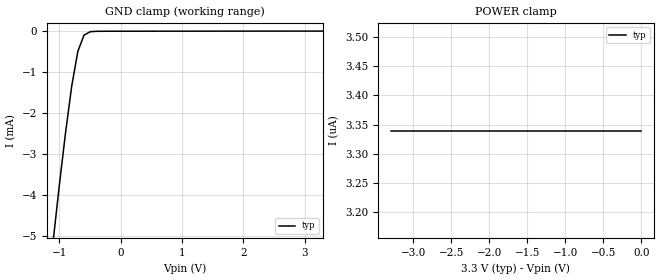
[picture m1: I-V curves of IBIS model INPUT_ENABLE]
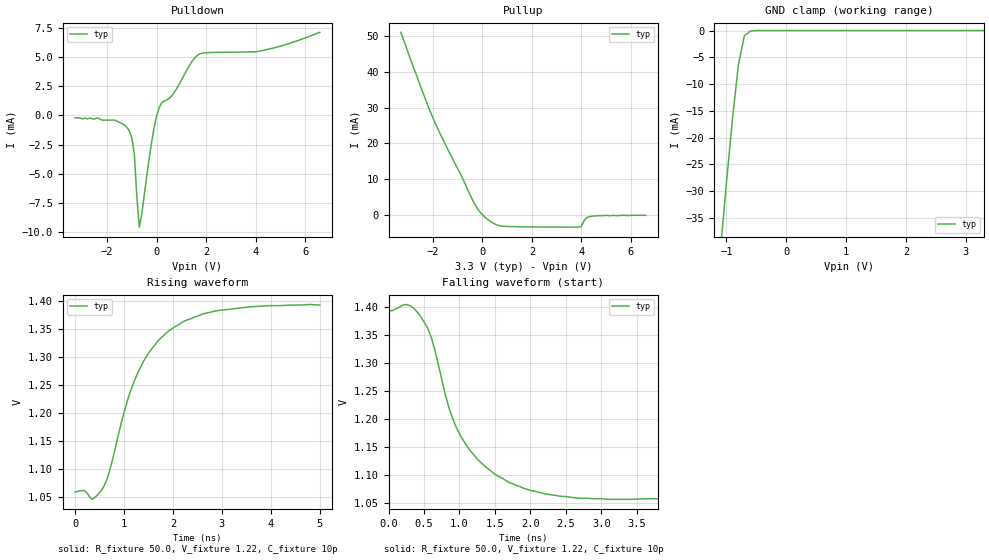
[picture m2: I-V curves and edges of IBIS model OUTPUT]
|   Texas Instruments Incorporated
|   Data Transmissions Products
|   IBIS Model for SN65LVDS389
|   38DBT TSSOP Package
[IBIS Ver]   2.1
[Comment char]   |_char
[File name]   lvds389.ibs
[File Rev]   1.0
[Date]   12Jan00
[Source]   File originated at Texas Instruments Incorporated.
   Data Transmission Products Group.
[Notes]   Model revved in Nov02 to fix common-mode bug  -TMF-
[Disclaimer]
(C) Copyright Texas Instruments Incorporated 2000
   All rights reserved
  Texas Instruments Incorporated hereby grants the user of this IBIS
model a non-exclusive, nontransferable license to use this IBIS model
under the following terms.  Before using this IBIS model, the user
should read this license.  If the user does not accept these terms,
the IBIS model should be returned to Texas Instruments within 30 days.
  The user is granted this license only to use the IBIS model and
is not granted rights to sell, load, rent, lease or license the IBIS
model in whole or in part, or in modified form to anyone other than
user.  User may modify the IBIS model to suit its specific applications
but rights to derivative works and such modifications shall belong to
Texas Instruments.
  This IBIS model is provided on an "AS IS" basis and Texas Instruments
makes absolutely no warranty with respect to the information contained
herein.  TEXAS INSTRUMENTS DISCLAIMS AND CUSTOMER WAIVES ALL WARRANTIES,
EXPRESS OR IMPLIED, INCLUDING WARRANTIES OF MERCHANTABILITY OR FITNESS
FOR A PARTICULAR PURPOSE. The entire risk as to quality and performance
is with the Customer. ACCORDINGLY, IN NO EVENT SHALL THE COMPANY BE LIABLE
FOR ANY DAMAGES, WHETHER IN CONTRACT OR TORT,INCLUDING ANY LOST PROFITS
OR OTHER INCIDENTAL, CONSEQUENTIAL, EXEMPLARY, OR PUNITIVE DAMAGES ARISING
OUT OF THE USE OR APPLICATION OF THE IBIS model provided in this package.
Further, Texas Instruments reserves the right to discontinue or make changes
without notice to any product herein to improve reliability, function, or
design. Texas Instruments does not convey any license under patent rights
or any other intellectual property rights, including those of third parties.
Contact Texas Instruments at ATTN:DATA TRANSMISSIONS
Thomas Fisher 12500 TI Boulevard, M/S 8710  Dallas, Texas 75243
[Copyright]   Copyright 2000, Texas Instruments, All Rights Reserved
[Component]   LVDS389DGG
[Manufacturer]  Texas Instruments Incorporated
[Package]
|   typ   min   max
R_pkg   0.040   0.035   0.047
L_pkg   2.433nH   1.956nH   3.508nH
C_pkg   0.451pF   0.362pF   0.635pF
[Pin]   signal_name   model_name   R_pin   L_pin   C_pin
1   GND   GND   0.047   3.508n   0.598p
2   VCC   POWER   0.047   3.231n   0.634p
3   GND   GND   0.046   2.932n   0.570p
4   ENA   INPUT_ENABLE   0.043   2.459n   0.459p
5   A1A   INPUT_ENABLE   0.035   2.103n   0.387p
6   A2A   INPUT_ENABLE   0.036   2.005n   0.369p
7   A3A   INPUT_ENABLE   0.035   1.956n   0.365p
8   A4A   INPUT_ENABLE   0.036   1.965n   0.364p
9   GND   GND   0.036   1.965n   0.363p
10   VCC   POWER   0.036   1.974n   0.362p
11   GND   GND   0.036   1.965n   0.362p
12   B1A   INPUT_ENABLE   0.036   1.965n   0.364p
13   B2A   INPUT_ENABLE   0.036   1.956n   0.365p
14   B3A   INPUT_ENABLE   0.036   2.005n   0.369p
15   B4A   INPUT_ENABLE   0.035   2.102n   0.387p
16   ENB   INPUT_ENABLE   0.043   2.459n   0.459p
17   GND   GND   0.046   2.932n   0.570p
18   VCC   POWER   0.047   3.231n   0.634p
19   GND   GND   0.047   3.508n   0.598p
20   B4Z   OUTPUT   0.047   3.508n   0.598p
21   B4Y   OUTPUT   0.047   3.231n   0.634p
22   B3Z   OUTPUT   0.046   2.932n   0.570p
23   B3Y   OUTPUT   0.043   2.459n   0.458p
24   B2Z   OUTPUT   0.035   2.103n   0.387p
25   B2Y   OUTPUT   0.036   2.005n   0.369p
26   B1Z   OUTPUT   0.035   1.956n   0.365p
27   B1Y   OUTPUT   0.036   1.965n   0.364p
28   NC   NC
29   NC   NC
30   NC   NC
31   A4Z   OUTPUT   0.036   1.965n   0.364p
32   A4Y   OUTPUT   0.036   1.956n   0.365p
33   A3Z   OUTPUT   0.036   2.004n   0.369p
34   A3Y   OUTPUT   0.035   2.102n   0.387p
35   A2Z   OUTPUT   0.043   2.459n   0.458p
36   A2Y   OUTPUT   0.046   2.932n   0.570p
37   A1Z   OUTPUT   0.047   3.231n   0.635p
38   A1Y   OUTPUT   0.047   3.508n   0.598p
[Diff_pin]   inv_pin   vdiff   tdelay_typ   tdelay_min   tdelay_max
| The 'xY' pin is Diff_pin and the 'xZ' pin is the inv_pin
21   20   NA   0 0 0
23   22   NA   0 0 0
25   24   NA   0 0 0
27   26   NA   0 0 0
32   31   NA   0 0 0
34   33   NA   0 0 0
36   35   NA   0 0 0
38   37   NA   0 0 0
| Models and submodels in the file (2): INPUT_ENABLE (Input), OUTPUT (3-state)
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|   Driver Input / Enable Model
[Model]   INPUT_ENABLE
Model_type   Input
|Signals   A1A,A2A,A3A,A4A,B1A,B2A,B3A,B4A
|   ENA,ENB,ENC,END
Vinh = 2.0
Vinl = 0.8
|   typ   min   max
C_comp   1.0pF   NA   NA
|   typ   min   max
[Temperature Range]   25.0   NA   NA
[Voltage range]   3.3V   3.0V   3.6V
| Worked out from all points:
|   GND clamp passes 1 mA (typ) near -0.76 V on its own axis
[GND_clamp]
|   Voltage   I(typ)   I(min)   I(max)
-3.3V     -43.1mA    NA         NA
-1.1V     -5.08mA    NA         NA
-1V       -3.73mA    NA         NA
-900mV    -2.47mA    NA         NA
-800mV    -1.34mA    NA         NA
-700mV    -493uA     NA         NA
-600mV    -98.5uA    NA         NA
-500mV    -13.3uA    NA         NA
3.3V      3.34uA     NA         NA
[Power_clamp]
| Note that the[POWER_clamp]voltage table is referenced to Vcc
| and is calculated using Vtable=Vcc - Vmeasured.
|   Voltage   I(typ)   I(min)   I(max)
-3.3V     3.34uA     NA         NA
-2.7V     3.34uA     NA         NA
-2V       3.34uA     NA         NA
-800mV    3.34uA     NA         NA
0V        3.34uA     NA         NA
|   Driver Output  MODEL
[Model]   OUTPUT
Model_type   3-state
| Signals   A1Y,A1Z,A2Y,A2Z,A3Y,A3Z,A4Y,A4Z,B1Y,B1Z,B2Y,B2Z,B3Y,B3Z,B4Y,B4Z
Vmeas = 1.2V   |Reference voltage for timing measurements
Cref = 10pF   |Timing specification test load capacitance value
Rref = 50   |Note: 50 Ohm load; single ended configuration
Vref = 1.20V   |Timing specification test load voltage
| variable   typ   min   max
C_comp   1.0pF   NA   NA
|   typ   min   max
[Temperature Range]   25.0   NA   NA
[Voltage range]   3.3V   3.0V   3.6V
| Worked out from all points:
|   slope of the pulldown table from 0 to 0.495 V, typ, clamps not added: 335 ohm
|   slope of the pullup table from 0 to 0.495 V, typ, clamps not added: 192 ohm
|   GND clamp passes 1 mA (typ) near -0.70 V on its own axis
|   rising waveform, R_fixture 50.0, V_fixture 1.22, C_fixture 10p: 20-80 % time 879ps typ, NA min, NA max; typ from 1.06 V to 1.39 V
|   falling waveform, R_fixture 50.0, V_fixture 1.22, C_fixture 10p: 20-80 % time 611ps typ, NA min, NA max; typ from 1.39 V to 1.06 V
[Pulldown]
|   Voltage   I(typ)   I(min)   I(max)
-3.3V     -200uA     NA         NA
-1.7V     -400uA     NA         NA
-1.1V     -1.34mA    NA         NA
-900mV    -3.37mA    NA         NA
-800mV    -6.98mA    NA         NA
-700mV    -9.59mA    NA         NA
-200mV    -2.26mA    NA         NA
100mV     664uA      NA         NA
700mV     1.94mA     NA         NA
1.6V      5.08mA     NA         NA
4.3V      5.58mA     NA         NA
6.6V      7.14mA     NA         NA
[Pullup]
|   Voltage   I(typ)   I(min)   I(max)
| Note that the[Pullup]voltage table is referenced to Vcc
| and is calculated using Vtable=Vcc - Vmeasured.
-3.3V     51mA       NA         NA
-2.2V     30.4mA     NA         NA
-1.7V     22.5mA     NA         NA
-300mV    2.87mA     NA         NA
-100mV    817uA      NA         NA
300mV     -1.72mA    NA         NA
900mV     -3.18mA    NA         NA
3.9V      -3.41mA    NA         NA
4V        -3.21mA    NA         NA
4.2V      -820uA     NA         NA
4.4V      -370uA     NA         NA
6.6V      -100uA     NA         NA
[GND_clamp]
|   Voltage   I(typ)   I(min)   I(max)
| Outputs in High Impedance (off)
-3.3V     -347mA     NA         NA
-1.1V     -41.1mA    NA         NA
-1V       -28.5mA    NA         NA
-900mV    -16.6mA    NA         NA
-800mV    -6.42mA    NA         NA
-700mV    -997uA     NA         NA
-600mV    -101uA     NA         NA
3.3V      -64pA      NA         NA
[POWER_clamp]
|   Voltage   I(typ)   I(min)   I(max)
| Note that the [POWER_clamp] voltage table is referenced to Vcc
| and is calculated using Vtable = Vcc - Vmeasured.
| Outputs in Tri-state.
-3.3V     0A         NA         NA
0V        0A         NA         NA
[Ramp]
|   typ   min   max
dV/dt_r   0.202/870ps   NA   NA
dV/dt_f   0.199/749ps   NA   NA
R_load = 50ohm
[Rising Waveform]
R_fixture = 50.0
V_fixture = 1.22
C_fixture = 10p
L_fixture = 0n
|   V(typ)   V(min)   V(max)
0s        1.059V     NA         NA
350ps     1.046V     NA         NA
550ps     1.063V     NA         NA
700ps     1.095V     NA         NA
1.05ns    1.216V     NA         NA
1.25ns    1.265V     NA         NA
1.5ns     1.306V     NA         NA
1.9ns     1.345V     NA         NA
2.9ns     1.382V     NA         NA
5ns       1.392V     NA         NA
[Falling Waveform]
R_fixture = 50.0
V_fixture = 1.22
C_fixture = 10p
L_fixture = 0n
|   V(typ)   V(min)   V(max)
0s        1.393V     NA         NA
250ps     1.404V     NA         NA
450ps     1.383V     NA         NA
600ps     1.346V     NA         NA
850ps     1.22V      NA         NA
1ns       1.173V     NA         NA
1.25ns    1.128V     NA         NA
1.7ns     1.086V     NA         NA
2.7ns     1.058V     NA         NA
5ns       1.061V     NA         NA
